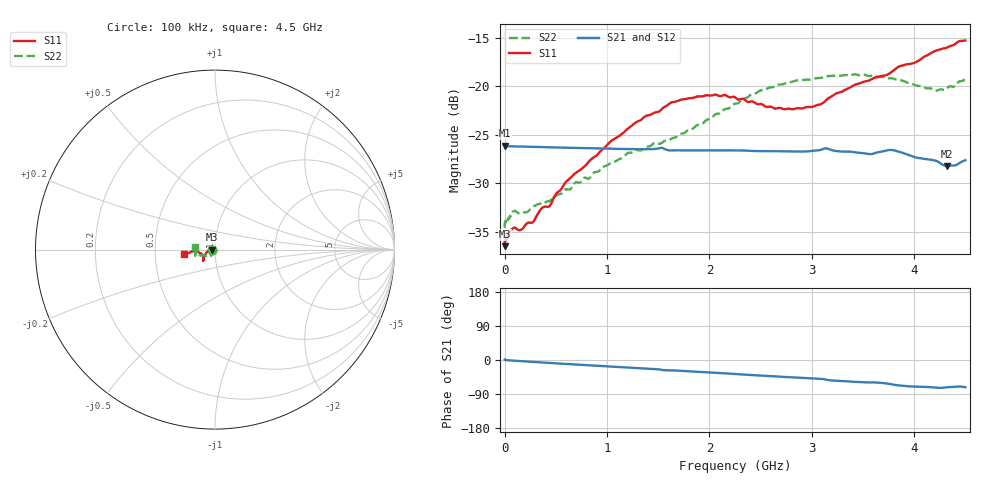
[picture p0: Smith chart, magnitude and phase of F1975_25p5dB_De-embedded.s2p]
! Integrated Device Technology
! Corporate Headquarters
! 6024 Silver Creek Valley Road
! San Jose, CA 95138  USA
! Phone:  1-408-284-8200
! Toll Free:  1-800-223-1366
! Webpage:  http://www.idt.com/
! Timing and RF Division
! 515 Groton Road, Suite 102
! Westford, MA 01886-6024
! Device:  F1975
! Description: 6-bit, 75 ohm, 0.5 dB Digital Step Attenuator
! Frequency:  5.0 MHz -  3.00 GHz
! Package:  4x4 mm QFN Plastic Package: 20 pin
! Ports:  2 RF, 11 DC
!  Pin  1  = D5 (16 dB)
!  Pin  2  = RF1  =  Port 1
!  Pin  3  = Serial Data In (DATA)
!  Pin  4  = Serial Clock (CLK)
!  Pin  5  = Serial Latch Enable (LE)
!  Pin  6  = VDD
!  Pin  7  = NC
!  Pin  8  = NC
!  Pin  9  = NC
!  Pin 10  = GND
!  Pin 11  = GND
!  Pin 12  = NC
!  Pin 13  = VMODE
!  Pin 14  = RF2  =  Port 2
!  Pin 15  = D4 (8 dB)
!  Pin 16  = D3 (4 dB)
!  Pin 17  = D2 (2 dB)
!  Pin 18  = NC
!  Pin 19  = D1 (1 dB)
!  Pin 20  = D0 (0.5 dB)
! State:  51
! Atten State:  25.5 dB
! Voltage:  +3.30 Volts
! Current:  0.561 mA
! Data:  The device was measured on a F1975 evaluation board which has
!  individual transmission lines to the RF pins.  Data was collected
!  using a calibrated network analyzer.  The evaluation board was
!  de-embedded using Automatic Fixture Removal (AFR).
!  The reference plane is the edge of the package pin.
! Misc:
!  Action Tracker AT0415
! Date Measured:  2018-02-08
! Date:  2018-03-26  MJV
! Note:
!  Integrated Device Technology supplies this data as a sample of measured
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# GHz S dB R 75
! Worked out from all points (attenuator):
!   291 points, 100 kHz to 4.5 GHz, reference 75 ohm
!   highest |S21| = -26.12 dB at 400 kHz (marker M1); lowest = -28.2 dB at 4.32 GHz (marker M2)
!   lowest |S11| = -36.5 dB at 100 kHz (marker M3), VSWR 1.03, Z = 72.8 + j0.00541 ohm
!   |S11| at or under -10 dB: start of sweep to end of sweep
!   |S22| runs from -34.5 to -18.8 dB; largest |S21 - S12| = 0.00019
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0.0001  -36.49 179.9  -26.13 1.1  -26.11 1.2  -34.49 -179.1
0.0004  -36.35 -179.2  -26.12 1.1  -26.13 1.1  -34.40 -178.8
0.006  -35.93 -178.4  -26.15 0.3  -26.16 0.3  -33.98 -177.7
0.08  -34.64 -176.3  -26.19 -1.6  -26.19 -1.5  -32.93 -168.6
0.16  -34.80 -176.9  -26.22 -3.0  -26.22 -3.0  -33.16 -158.1
0.28  -33.99 179.7  -26.25 -5.1  -26.25 -5.1  -32.39 -149.2
0.36  -32.59 179.9  -26.27 -6.4  -26.27 -6.5  -32.03 -141.6
0.44  -32.36 -179.3  -26.29 -7.8  -26.29 -7.8  -31.87 -135.7
0.6  -29.84 -175.6  -26.33 -10.4  -26.33 -10.4  -30.60 -130.2
0.76  -28.45 -168.8  -26.37 -13.0  -26.37 -13.0  -29.64 -126.6
1.28  -23.74 -152.4  -26.48 -21.2  -26.48 -21.2  -26.59 -123.2
1.52  -22.51 -144.4  -26.35 -25.1  -26.35 -25.1  -25.92 -129.8
1.62  -21.70 -142.7  -26.62 -27.3  -26.61 -27.3  -25.45 -133.3
1.88  -21.06 -138.7  -26.60 -30.7  -26.60 -30.7  -24.00 -145.9
2.26  -21.21 -137.7  -26.61 -37.1  -26.61 -37.1  -21.79 -156.9
2.64  -22.31 -147.1  -26.70 -43.2  -26.69 -43.2  -20.02 -158.8
3.02  -22.07 -163.6  -26.65 -48.8  -26.64 -48.9  -19.22 -159.8
3.42  -19.84 -175.1  -26.81 -57.7  -26.80 -57.7  -18.76 -164.4
3.76  -18.67 -175.6  -26.56 -63.1  -26.56 -63.1  -19.17 -170.0
4.2  -16.38 -172.6  -27.65 -72.5  -27.65 -72.6  -20.44 178.5
4.32  -16.01 -172.2  -28.22 -72.1  -28.21 -72.1  -20.22 176.3
4.5  -15.27 -172.2  -27.63 -71.8  -27.62 -71.8  -19.19 173.6
